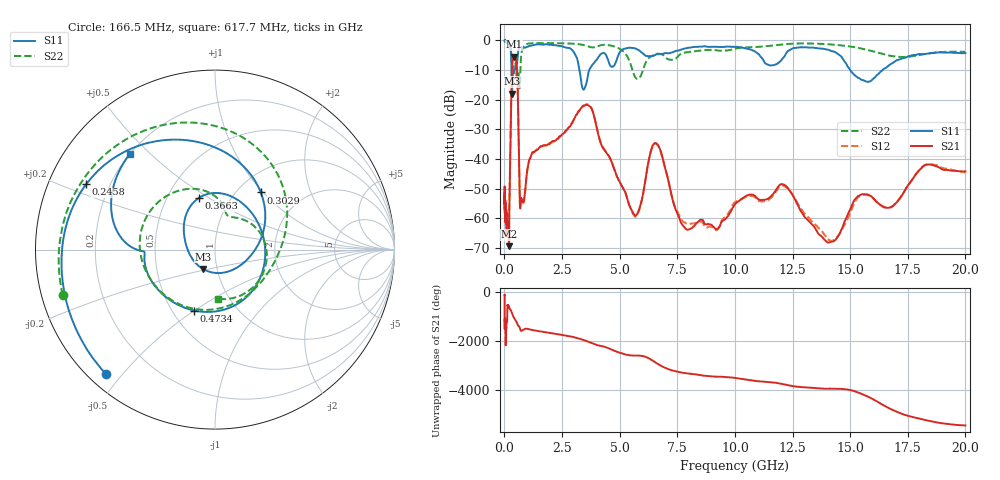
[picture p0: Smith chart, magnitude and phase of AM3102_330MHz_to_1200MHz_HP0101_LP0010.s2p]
! Date/Time: Tue, Sep 11, 2018 5:13 PM
! Network Analyzer: Agilent Technologies E8362B Rev: A.07.50.63
! Sweep from 0.010 to 20.000 GHz, 1601 Points, Sweep Type: LOG
! Power Supply: 4.949 V, 0.001 A
# Hz S DB R 50
!freq MagS11 AngS11 MagS21 AngS21 MagS12 AngS12 MagS22 AngS22
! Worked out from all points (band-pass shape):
!   1601 points, 10 MHz to 20 GHz, reference 50 ohm
!   highest |S21| = -5.46 dB at 416.5 MHz (marker M1); lowest = -69.4 dB at 200.4 MHz (marker M2)
!   |S21| within 3 dB of the highest: 334.6 MHz to 540.5 MHz (205.9 MHz wide, 47.1 % of centre)
!   lowest |S11| = -17.9 dB at 333.1 MHz (marker M3), VSWR 1.29, Z = 42.8 - j9.41 ohm
!   |S11| at or under -10 dB: 309.6 MHz to 444.8 MHz (135.2 MHz wide, 35.8 % of centre); 3.257 GHz to 3.682 GHz (425.2 MHz wide, 12.3 % of centre); 15.01 GHz to 16.4 GHz (1.399 GHz wide, 8.91 % of centre)
!   |S22| runs from -16.2 to -0.2 dB; largest |S21 - S12| = 0.0076
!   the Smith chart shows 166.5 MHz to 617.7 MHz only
!   S11 on the Smith chart (normalised r, x): 166.5 MHz: 0.05, -0.45; 245.8 MHz: 0.11, +0.24; 302.9 MHz: 1.27, +0.97; 366.3 MHz: 0.71, +0.45; 473.4 MHz: 0.64, -0.50; 617.7 MHz: 0.20, +0.43
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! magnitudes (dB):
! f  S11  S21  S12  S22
! 10 MHz  0.0  -54.8  -52.3  -0.2
! 35.55 MHz  0.0  -58.6  -58.9  -0.4
! 126.4 MHz  -0.4  -64.1  -64.8  -0.8
! 166.5 MHz  -0.7  -62.3  -65.7  -1.1
! 200.4 MHz  -1.2  -69.4  -62.7  -1.3
! 245.8 MHz  -1.9  -43.0  -42.8  -2.0
! 302.9 MHz  -7.8  -16.7  -16.7  -4.9
! 333.1 MHz  -17.9  -8.7  -8.7  -8.9
! 366.3 MHz  -10.4  -6.3  -6.3  -9.8
! 416.5 MHz  -11.1  -5.5  -5.5  -7.9
! 447.2 MHz  -9.9  -5.6  -5.7  -7.5
! 473.4 MHz  -8.9  -5.9  -5.9  -7.7
! 617.7 MHz  -2.9  -32.5  -32.6  -11.2
! 689.1 MHz  -2.3  -56.8  -56.6  -11.3
! 1.59 GHz  -1.4  -35.7  -35.8  -0.9
! 3.651 GHz  -10.7  -21.9  -21.7  -2.0
! 5.652 GHz  -2.6  -59.0  -59.3  -12.1
! 6.549 GHz  -4.9  -34.6  -34.8  -4.8
! 7.958 GHz  -2.5  -63.9  -62.0  -3.9
! 12.03 GHz  -6.5  -48.5  -49.0  -1.4
! 14.14 GHz  -3.4  -68.0  -67.6  -1.3
! 20 GHz  -4.3  -44.2  -44.6  -3.8
